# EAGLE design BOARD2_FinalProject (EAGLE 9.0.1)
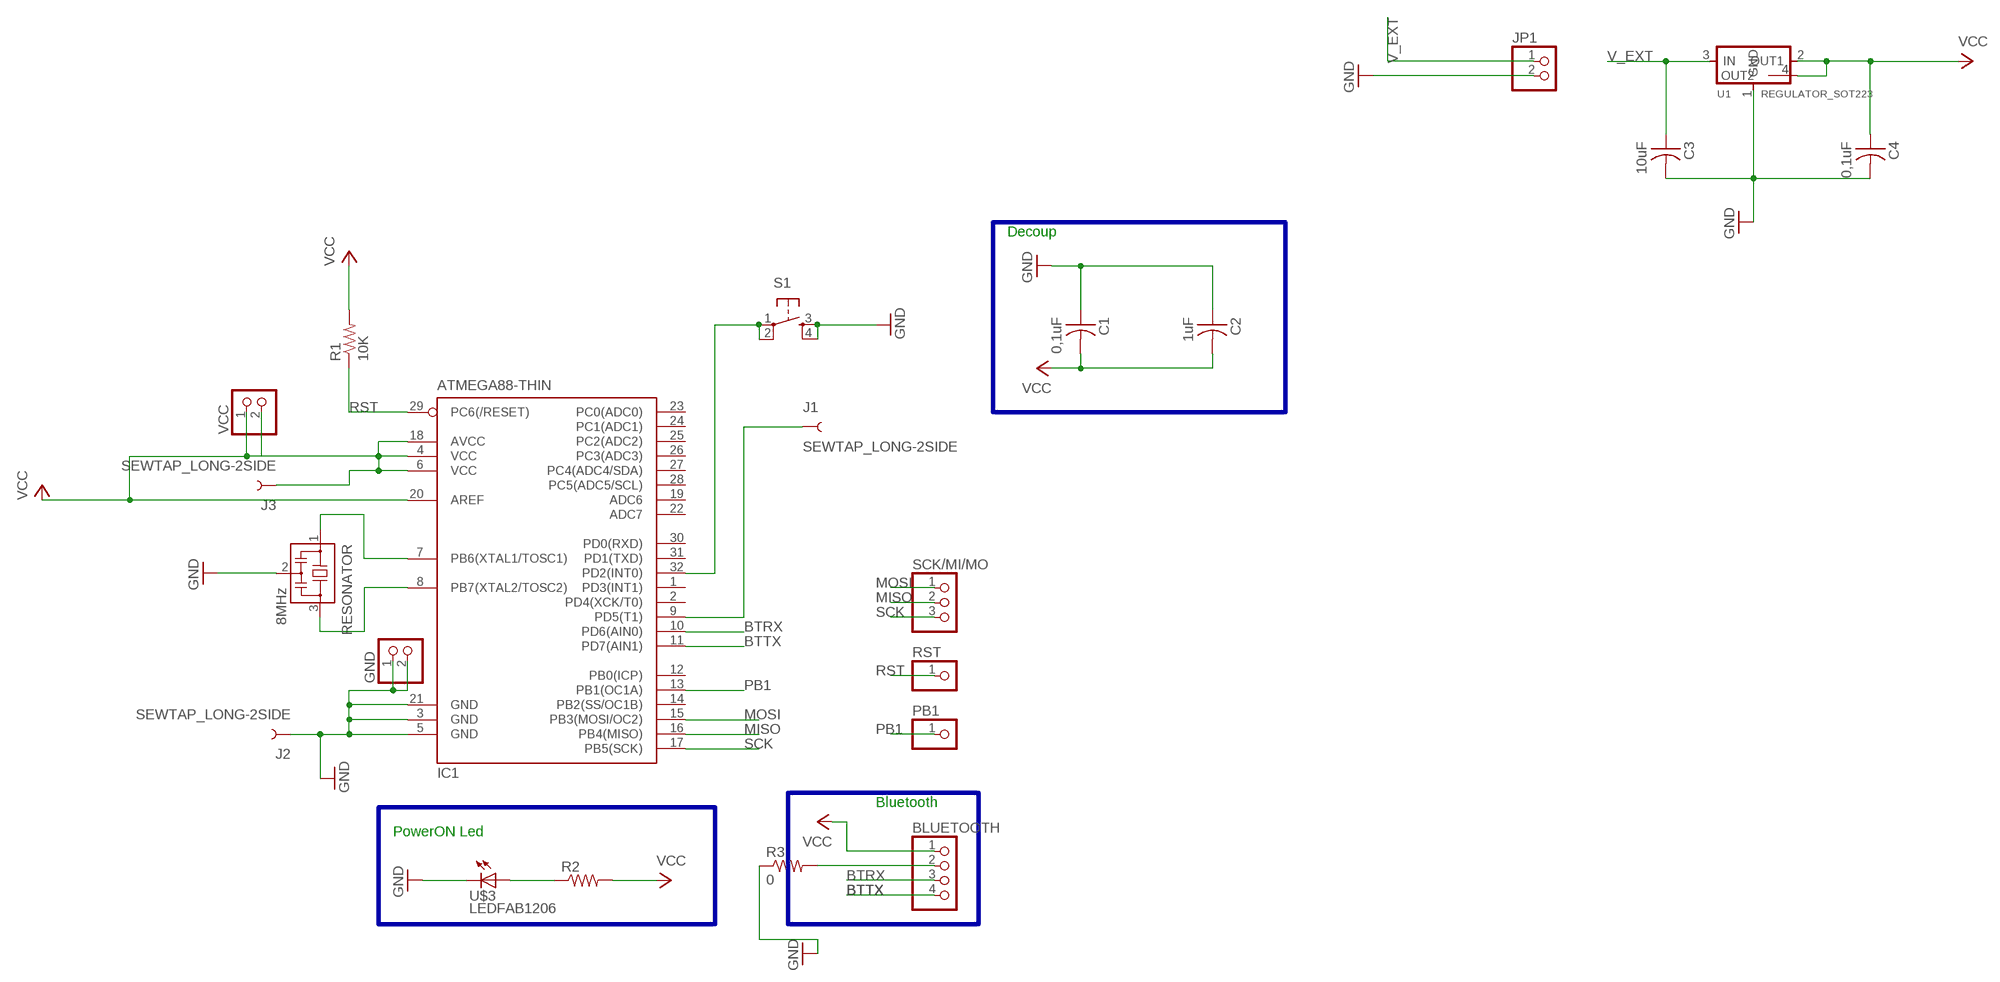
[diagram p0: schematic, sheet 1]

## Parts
BLUETOOTH  PINHD-1X4  [1X04]
C1  0,1uF  CAP-US1206FAB  [C1206FAB]
C2  1uF  CAP-US1206FAB  [C1206FAB]
C3  10uF  CAP-US1206FAB  [C1206FAB]
C4  0,1uF  CAP-US1206FAB  [C1206FAB]
GND  PINHD-1X2  [1X02]
IC1  ATMEGA88-THIN  [TQFP32-08THIN]
J1  SEWTAP_LONG-2SIDE  [PETAL-LONG-1-2SIDE]
J2  SEWTAP_LONG-2SIDE  [PETAL-LONG-1-2SIDE]
J3  SEWTAP_LONG-2SIDE  [PETAL-LONG-1-2SIDE]
JP1  PINHD-1X2  [1X02]
PB1  PINHD-1X1  [1X01]
R1  10K  RES-US1206FAB  [R1206FAB]
R2  RES-US1206FAB  [R1206FAB]
R3  0  RES-US1206FAB  [R1206FAB]
RESONATOR  8MHz  RESONATOR  [EFOBM]
RST  PINHD-1X1  [1X01]
S1  6MM_SWITCH6MM_SWITCH  [6MM_SWITCH]
SCK/MI/MO  PINHD-1X3  [1X03]
U1  REGULATOR_SOT223  [SOT223]
U$3  LEDFAB1206  [LED1206FAB]
VCC  PINHD-1X2  [1X02]

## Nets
BTRX: BLUETOOTH.3 IC1.10(PD6(AIN0))
BTTX: BLUETOOTH.4 IC1.11(PD7(AIN1))
GND: C1.1 C2.1 C3.2 C4.2 GND.1 GND.2 IC1.3(GND) IC1.5(GND) IC1.21(GND) J2.1 JP1.2 R3.1 RESONATOR.2 S1.3(S) S1.4(S1) U1.1(GND) U$3.2(C)
MISO: IC1.16(PB4(MISO)) SCK/MI/MO.2
MOSI: IC1.15(PB3(MOSI/OC2)) SCK/MI/MO.1
N$1: BLUETOOTH.2 R3.2
N$2: IC1.32(PD2(INT0)) S1.1(P) S1.2(P1)
N$4: R2.1 U$3.1(A)
N$8: IC1.9(PD5(T1)) J1.1
N$11: IC1.8(PB7(XTAL2/TOSC2)) RESONATOR.3
N$12: IC1.7(PB6(XTAL1/TOSC1)) RESONATOR.1
PB1: IC1.13(PB1(OC1A)) PB1.1
RST: IC1.29(PC6(/RESET)) R1.1 RST.1
SCK: IC1.17(PB5(SCK)) SCK/MI/MO.3
V_EXT: C3.1 JP1.1 U1.3(IN)
VCC: BLUETOOTH.1 C1.2 C2.2 C4.1 IC1.4(VCC) IC1.6(VCC) IC1.18(AVCC) IC1.20(AREF) J3.1 R1.2 R2.2 U1.2(OUT1) U1.4(OUT2) VCC.1 VCC.2
Unconnected: IC1.1(PD3(INT1)) IC1.2(PD4(XCK/T0)) IC1.12(PB0(ICP)) IC1.14(PB2(SS/OC1B)) IC1.19(ADC6) IC1.22(ADC7) IC1.23(PC0(ADC0)) IC1.24(PC1(ADC1)) IC1.25(PC2(ADC2)) IC1.26(PC3(ADC3)) IC1.27(PC4(ADC4/SDA)) IC1.28(PC5(ADC5/SCL)) IC1.30(PD0(RXD)) IC1.31(PD1(TXD))

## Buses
B$1
B$2
B$3

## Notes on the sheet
- Decoup
- Bluetooth
- PowerON Led

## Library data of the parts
BLUETOOTH = pinhead:PINHD-1X4: PIN HEADER
C1-C4 = 1_fab:CAP-US
GND JP1 VCC = pinhead:PINHD-1X2: PIN HEADER
IC1 = fab:ATMEGA88-THIN
J1-J3 = LilyPad-Wearables:SEWTAP: SparkFun LilyPad Sew Taps
PB1 RST = pinhead:PINHD-1X1: PIN HEADER
R1 R2 = fab:RES-US: Resistor (US Symbol)
R3 = 1_fab:RES-US: Resistor (US Symbol)
RESONATOR = fab:RESONATOR
S1 = 1_fab:6MM_SWITCH: OMRON SWITCH
SCK/MI/MO = pinhead:PINHD-1X3: PIN HEADER
U1 = 1_fab:REGULATOR_SOT223
U$3 = fab:LED: LED

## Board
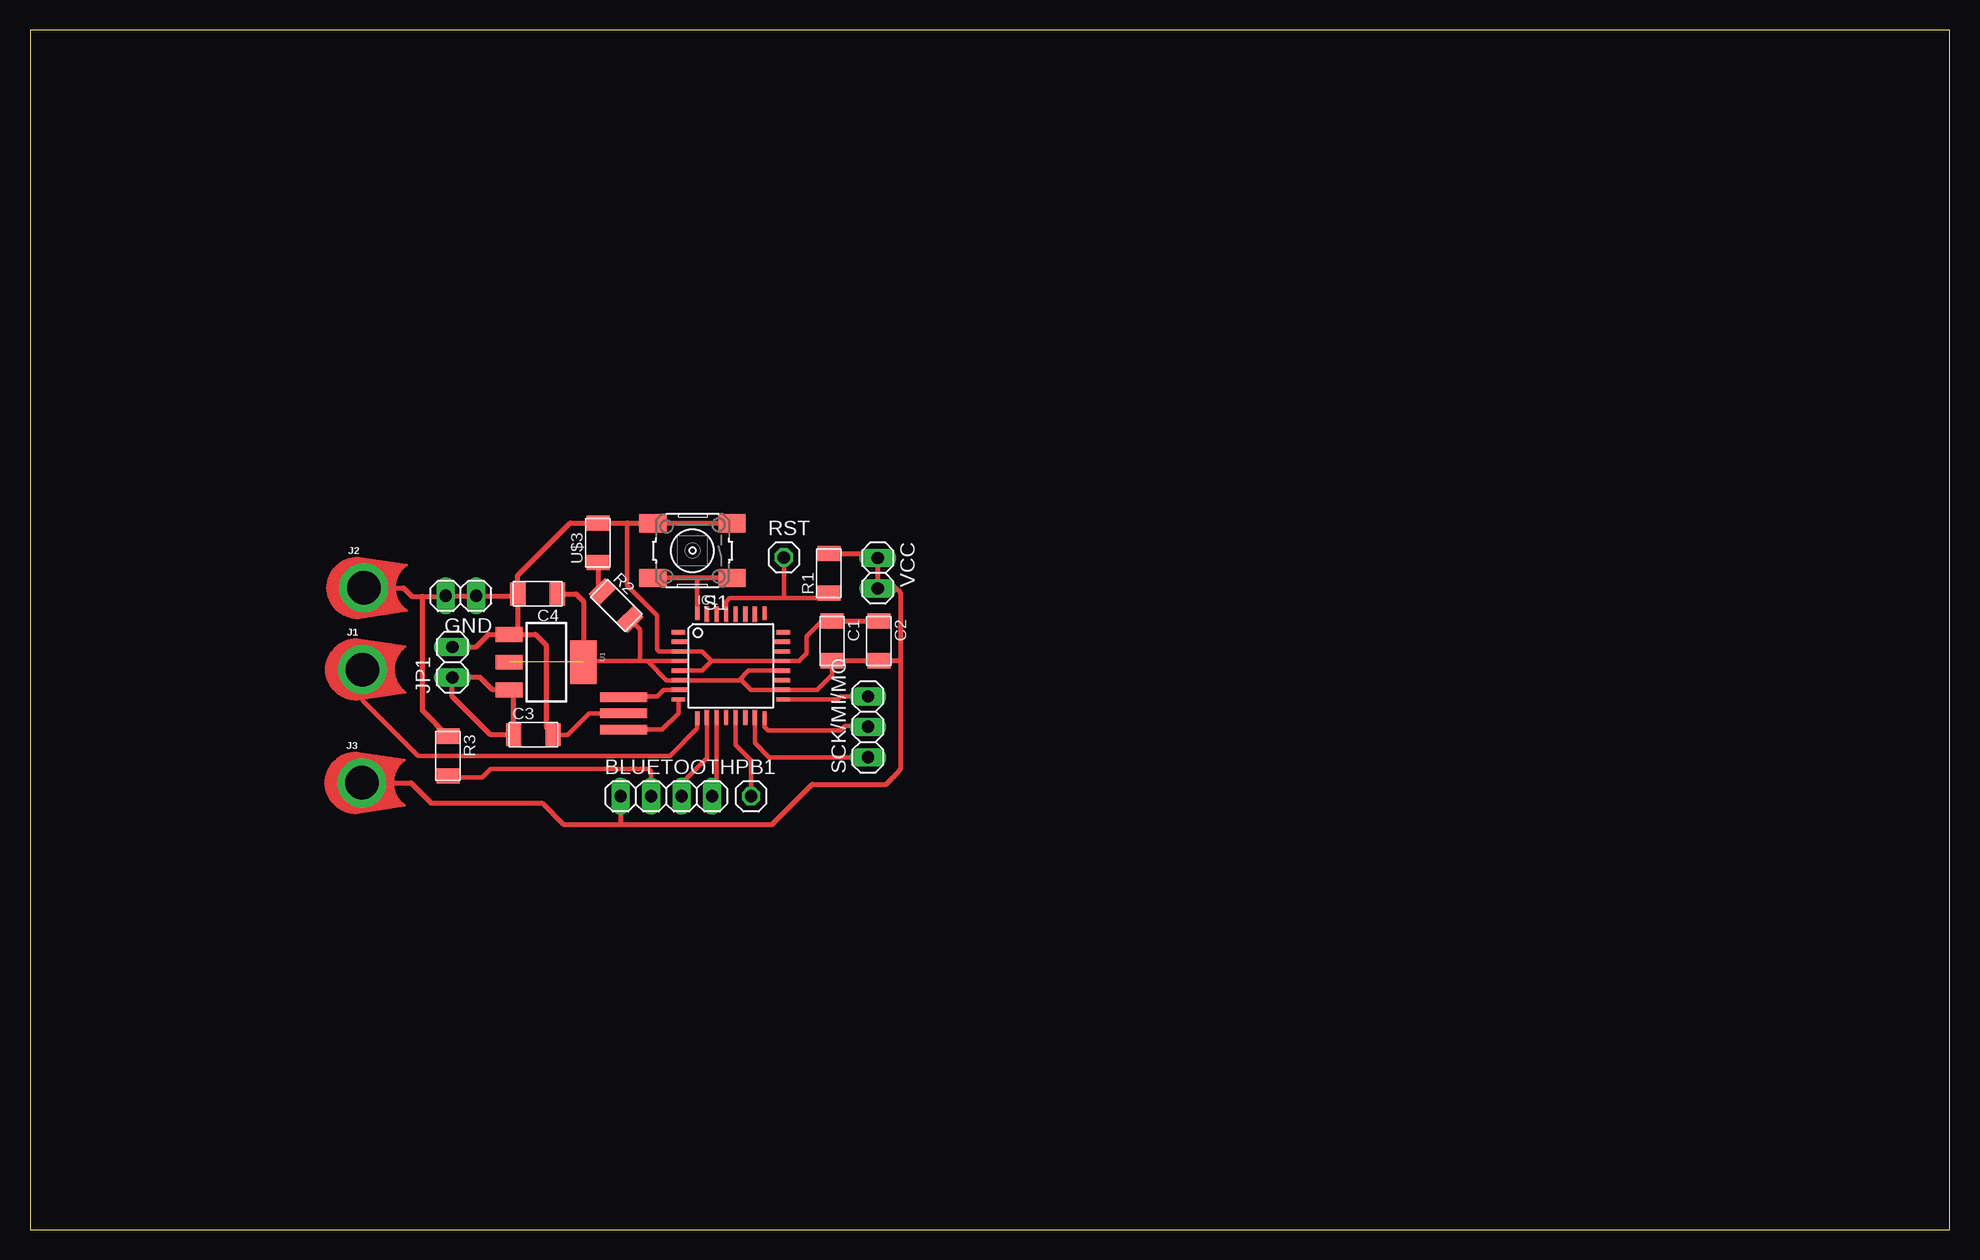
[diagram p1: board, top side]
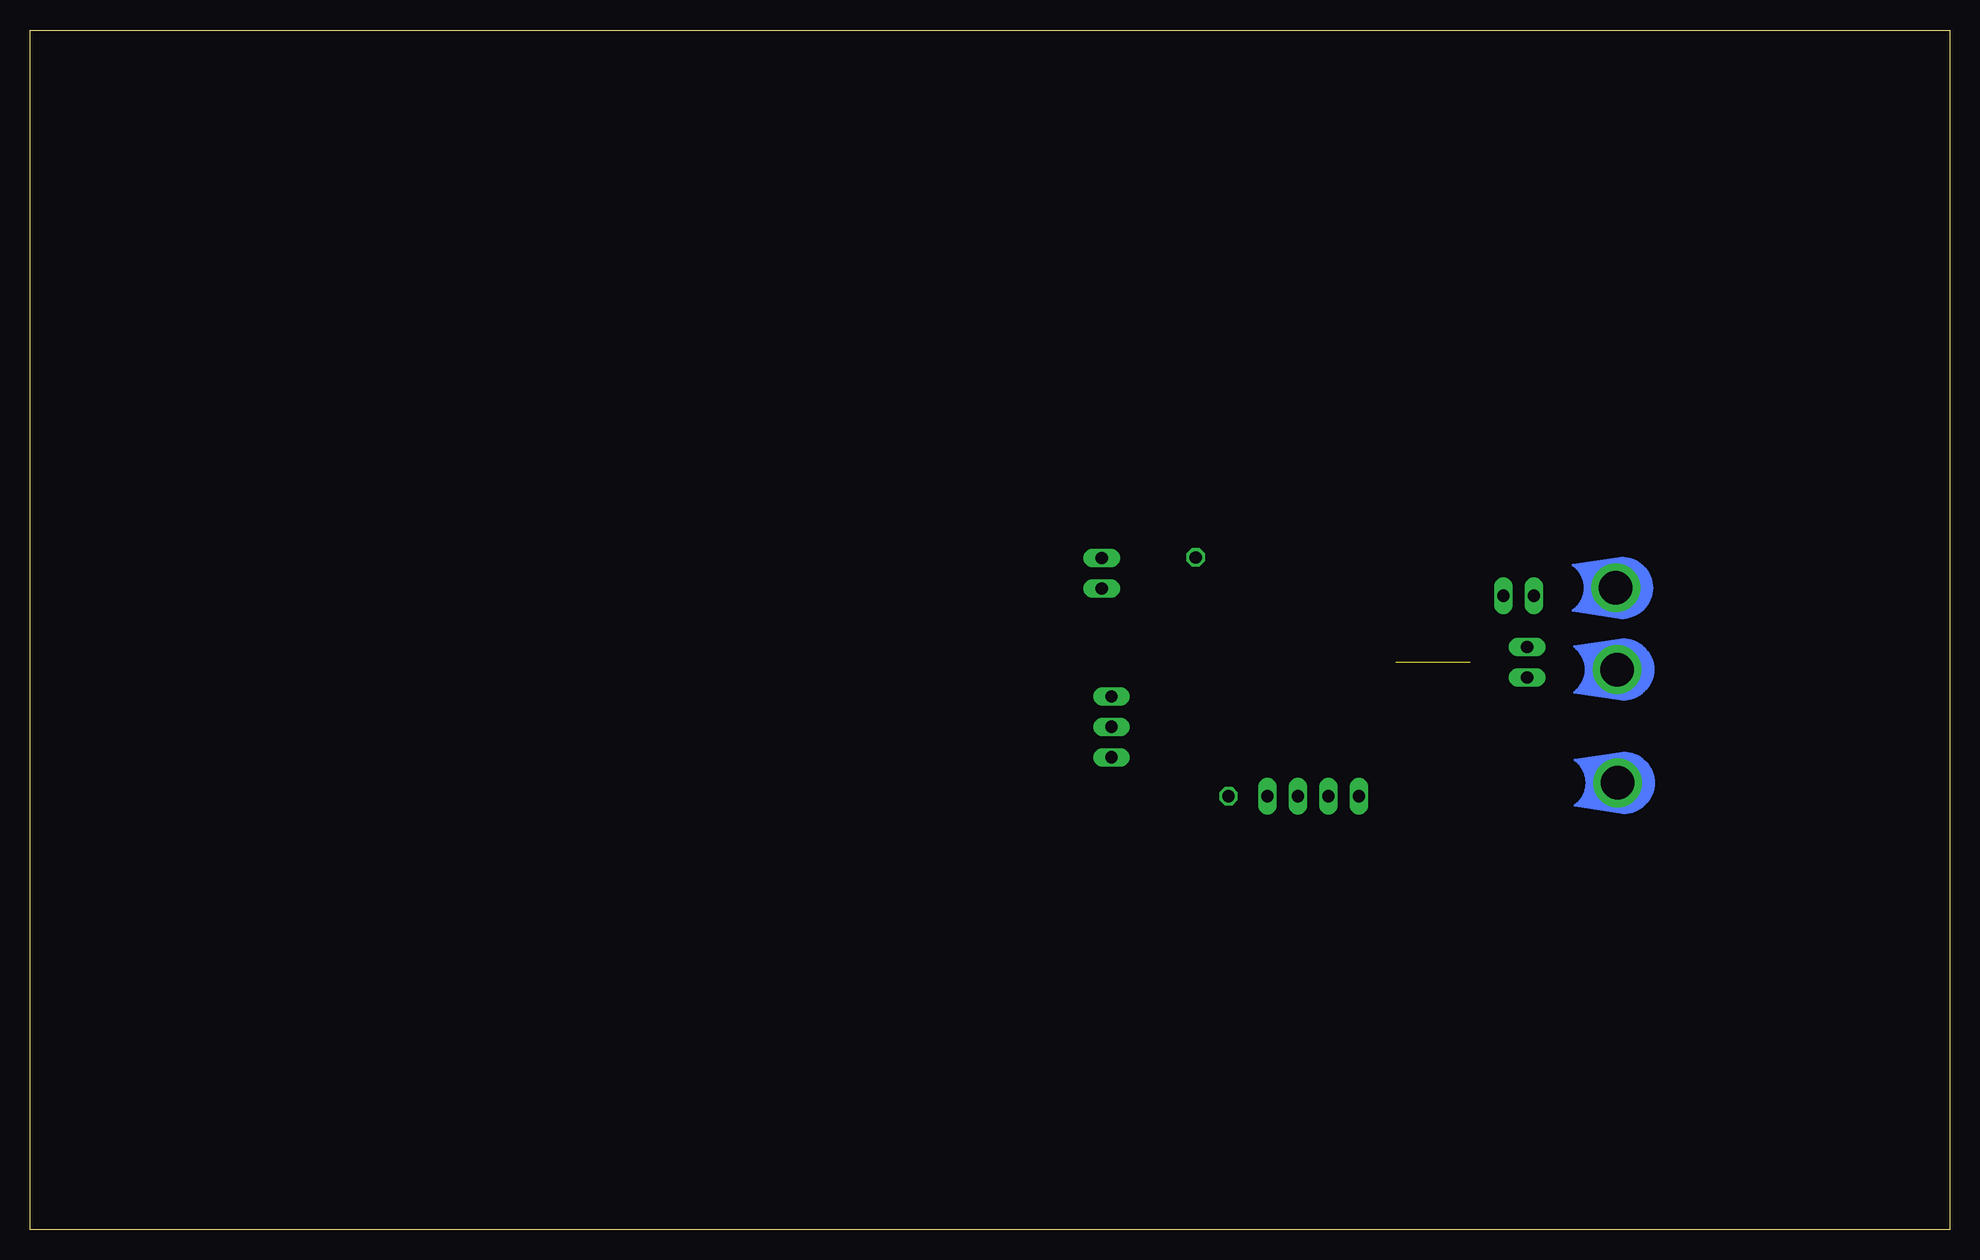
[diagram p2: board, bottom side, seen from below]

Size 160 x 100 mm. Coordinates in mm from the lower left corner, seen from the top.
Outline: 0,0 160,0 160,100 0,100 0,0
Copper layers (1*16): Top 0.035mm / dielectric 1.5mm / Bottom 0.035mm
Design rules "default": minimum track width 6mil, minimum drill 0.35mm, track to track 6mil, track to pad 6mil, pad to pad 6mil, via to via 6mil, smd to smd 6mil, copper to edge 40mil, drill to drill 6mil, minimum pad ring 10mil, minimum via ring 8mil, stop-mask expansion 4mil, vias tented up to drill 0mil, thermal gap 10mil

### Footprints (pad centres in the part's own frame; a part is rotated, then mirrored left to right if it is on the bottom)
1X04 = drill 1.016 long: 1 -3.81,0; 2 -1.27,0; 3 1.27,0; 4 3.81,0
C1206FAB = smd 1.27 x 1.905: 1 -1.651,0; 2 1.651,0
1X02 = drill 1.016 long: 1 -1.27,0; 2 1.27,0
TQFP32-08THIN = smd 1.118 x 0.356: 1 -4.369,2.8; 8 -4.369,-2.8; 17 4.369,-2.8; 24 4.369,2.8 | smd 1.27 x 0.356: 2 -4.293,2; 3 -4.293,1.2; 4 -4.293,0.4; 5 -4.293,-0.4; 6 -4.293,-1.2; 7 -4.293,-2; 18 4.293,-2; 19 4.293,-1.2; 20 4.293,-0.4; 21 4.293,0.4; 22 4.293,1.2; 23 4.293,2 | smd 0.356 x 1.118: 9 -2.8,-4.369; 16 2.8,-4.369; 25 2.8,4.369; 32 -2.8,4.369 | smd 0.356 x 1.27: 10 -2,-4.293; 14 1.2,-4.293; 15 2,-4.293; 26 2,4.293; 27 1.2,4.293; 31 -2,4.293 | smd 0.35 x 1.27: 11 -1.2,-4.293; 12 -0.4,-4.293; 13 0.4,-4.293; 28 0.4,4.293; 29 -0.4,4.293; 30 -1.2,4.293
PETAL-LONG-1-2SIDE = drill 2.794 pad 4.064: 1 0.03,0
1X01 = drill 1.016 octagon: 1 0,0
R1206FAB = smd 1.27 x 1.905: 1 -1.651,0; 2 1.651,0
EFOBM = smd 0.8 x 3.9: 1 -1.35,0; 2 0,0; 3 1.35,0
6MM_SWITCH = smd 2.286 x 1.524: 1 -3.302,2.286; 2 3.302,2.286; 3 -3.302,-2.286; 4 3.302,-2.286
1X03 = drill 1.016 long: 1 -2.54,0; 2 0,0; 3 2.54,0
SOT223 = smd 1.219 x 2.235: 1 -2.311,-3.099; 2 0,-3.099; 3 2.311,-3.099 | smd 3.6 x 2.2: 4 0,3.099
LED1206FAB = smd 1.27 x 1.905: 1 -1.651,0; 2 1.651,0

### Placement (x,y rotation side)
BLUETOOTH  53.04,36.12 0 top
C1  66.85,49.07 270 top
C2  70.76,49.07 270 top
C3  41.96,41.25 0 top
C4  42.32,52.98 180 top
GND  35.92,52.83 180 top
IC1  58.42,46.99 0 top
J1  27.69,46.69 0 top
J2  27.79,53.49 0 top
J3  27.64,37.24 0 top
JP1  35.2,47.29 90 top
PB1  60.1,36.12 0 top
R1  66.6,54.71 90 top
R2  48.87,52.02 315 top
R3  34.85,39.47 270 top
RESONATOR  49.48,43.03 270 top
RST  62.84,56.03 0 top
S1  55.22,56.59 180 top
SCK/MI/MO  69.85,41.91 90 top
U1  43.03,47.29 270 top
U$3  47.35,57.25 90 top
VCC  70.66,54.71 270 top

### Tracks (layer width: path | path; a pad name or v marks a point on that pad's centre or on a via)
BTRX
  Top 0.356: IC1.10 56.42,39.3 54.3,37.19 BLUETOOTH.3
BTTX
  Top 0.356: BLUETOOTH.4 57.22,36.49 IC1.11
GND
  Top 0.356: 56.8,47.39 56,48.19 IC1.3 52.45,48.19 52.27,48.36 52.27,51.21 49.78,53.7 49.78,58.9 | 56.8,47.39 IC1.21 64.1,47.39 64.72,48.01 64.72,49.43 66.02,50.72 C1.1 | IC1.5 56,46.59 56.8,47.39 | RESONATOR.2 46.58,43.03 45.34,41.78 44.81,41.25 C3.2
  Top 0.406: C4.2 40.66,54.53 45.03,58.9 U$3.2 49.78,58.9 51.89,58.9 S1.4 S1.3 | 40.54,49.61 U1.1 38.23,49.61 37.19,48.56 JP1.2 | 40.54,49.61 42.14,49.61 43.03,48.72 43.03,41.83 C3.2 | C4.2 40.66,49.73 40.54,49.61 | 32.72,52.78 34.59,52.78 GND.2 GND.1 40.51,52.83 C4.2 | R3.1 32.72,43.26 32.72,52.78 | 32.72,52.78 31.85,52.78 31.14,53.49 J2.1 | C1.1 C2.1
MISO
  Top 0.356: IC1.16 61.22,41.9 61.52,41.6 67.56,41.6 67.92,41.96 69.8,41.96 SCK/MI/MO.2
MOSI
  Top 0.356: IC1.15 60.42,40.57 61.62,39.37 SCK/MI/MO.1
N$1
  Top 0.356: BLUETOOTH.2 51.77,38.2 51.56,38.41 38.41,38.41 37.69,37.69 35.2,37.69 34.96,37.94
  Top 0.406: 35.08,38.05 34.96,37.94 R3.2
N$2
  Top 0.356: IC1.32 55.62,54.1 55.83,54.3
  Top 0.406: S1.1 55.83,54.3 S1.2
N$4
  Top 0.406: U$3.1 47.35,53.54 R2.1
N$8
  Top 0.356: IC1.9 55.62,41.75 53.34,39.47 32.36,39.47 27.72,44.12 J1.1
N$11
  Top 0.356: RESONATOR.3 52.7,41.68 54.05,43.03 IC1.8
N$12
  Top 0.356: RESONATOR.1 49.55,44.45 52.27,44.45 52.81,44.99 IC1.7
PB1
  Top 0.356: IC1.13 58.82,40.39 60.1,39.12 PB1.1
RST
  Top 0.356: IC1.29 58.02,52.33 58.32,52.63 62.94,52.63 | RST.1 62.84,52.73 62.94,52.63 | R1.1 66.17,52.63 62.94,52.63
SCK
  Top 0.356: IC1.17 67.3,44.19 67.56,44.45 SCK/MI/MO.3
V_EXT
  Top 0.406: U1.3 38.58,44.98 37.54,46.02 JP1.1 35.2,44.45 38.41,41.25 C3.1 40.31,44.6 U1.3
VCC  (1 unrouted)
  Top 0.356: 62.58,46.58 62.59,46.59 IC1.20 59.91,46.58 59.11,45.79 | 51.66,47.39 51.56,47.3 53.07,45.79 IC1.6 59.11,45.79 | 51.66,47.39 IC1.4 | C1.2 66.85,46.23 65.61,44.99 IC1.18 60.1,44.99 59.3,45.79 59.11,45.79 | U1.4 46.22,47.39 49.43,47.39 50.85,47.39 | 50.85,47.39 51.66,47.39 | R2.2 50.85,50.04 50.85,47.39
  Top 0.406: C4.1 45.52,52.98 46.13,52.38 U1.4 | 49.23,34.7 BLUETOOTH.1 49.23,33.78 | 49.23,33.78 44.45,33.78 42.67,35.56 33.43,35.56 31.75,37.24 J3.1 | 49.23,33.78 61.87,33.78 65.2,37.11 71.35,37.11 71.89,37.65 72.54,38.41 72.54,47.3 | C2.2 71.83,47.42 | C2.2 71.35,47.65 | C1.2 C2.2 | R1.2 70.28,56.36 VCC.1 VCC.2 72.19,53.44 72.54,53.09 72.54,47.3 | C2.2 72.42,47.42 72.54,47.3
